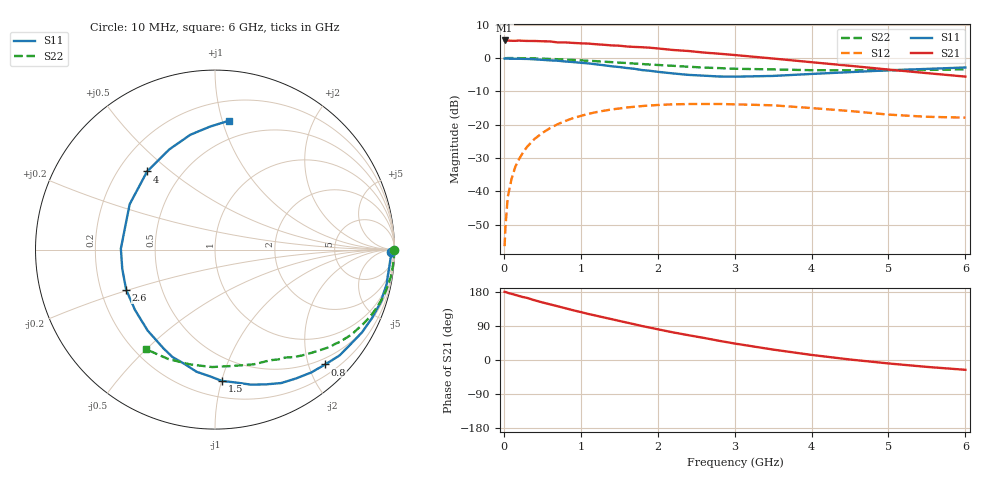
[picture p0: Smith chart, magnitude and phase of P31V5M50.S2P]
! SIEMENS Small Signal Semiconductors
! BFP181
! Si NPN RF Bipolar Junction Transistor in SOT143
! VCE = 1.5 V  IC = 0.5 mA
! Common Emitter S-Parameters:  March  1996
# GHz  S  MA  R  50
!  f  S11  S21  S12  S22
! GHz  MAG  ANG  MAG  ANG  MAG  ANG  MAG  ANG
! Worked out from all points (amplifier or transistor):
!   36 points, 10 MHz to 6 GHz, reference 50 ohm
!   highest |S21| = 5.3 dB at 10 MHz (marker M1)
!   |S21| within 3 dB of that: start of sweep to 2.291 GHz
!   unconditionally stable (mu >= 1): 3.69 GHz to end of sweep
!   at 250 MHz: K = 0.08, MSG = 16.8 dB, |S12| = -28.3 dB
!   at 1.4 GHz: K = 0.44, MSG = 9.6 dB, |S12| = -15.4 dB
!   at 6 GHz: K = 1.50, MAG = 2.0 dB, |S12| = -17.9 dB
!   S11 on the Smith chart (normalised r, x): 10 MHz: 75, -48; 800 MHz: 0.38, -2.29; 1.5 GHz: 0.32, -1.00; 2.6 GHz: 0.31, -0.20; 4 GHz: 0.32, +0.42; 6 GHz: 0.35, +1.05
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0.01  0.9812 -0.7  1.834 179.8  0.0015 89.0  0.9995 -0.2
0.02  0.9871 -1.4  1.833 179.6  0.0028 93.1  0.9925 -0.6
0.05  0.9793 -2.8  1.826 177.3  0.0081 89.5  0.998 -1.5
0.1  0.9757 -5.8  1.814 174.6  0.0153 85.8  0.9978 -2.8
0.15  0.9738 -8.7  1.811 171.8  0.0235 83.8  0.996 -4.2
0.25  0.9703 -14.5  1.813 166.0  0.0383 80.1  0.9928 -7.2
0.3  0.9694 -17.4  1.804 164.0  0.0462 77.7  0.992 -8.5
0.4  0.9546 -23.4  1.801 157.6  0.061 73.6  0.9854 -11.3
0.6  0.9214 -34.9  1.773 146.9  0.0886 65.2  0.9688 -16.9
0.8  0.8868 -46.2  1.712 136.6  0.1135 57.5  0.9475 -22.0
1.1  0.83 -63.6  1.646 121.4  0.1451 46.4  0.9081 -29.3
1.5  0.7326 -87.0  1.53 103.2  0.1747 33.0  0.8511 -38.1
1.9  0.6434 -111.7  1.427 85.4  0.1936 21.6  0.797 -45.5
2.2  0.5867 -129.8  1.319 72.9  0.2018 14.2  0.7635 -50.6
2.6  0.5431 -155.7  1.207 58.3  0.2041 5.3  0.7179 -56.9
3  0.5245 179.4  1.109 43.5  0.2017 -3.3  0.6896 -63.3
3.5  0.5384 152.0  0.982 27.5  0.1951 -11.4  0.6748 -71.3
4  0.5767 131.0  0.865 13.4  0.1773 -17.6  0.6562 -80.9
4.5  0.6136 114.5  0.764 1.3  0.1601 -22.3  0.6546 -91.4
5  0.6545 102.1  0.671 -9.1  0.1414 -23.2  0.6545 -102.2
5.5  0.686 92.3  0.593 -18.2  0.1312 -19.5  0.663 -113.3
6  0.7212 84.0  0.526 -25.9  0.1273 -15.2  0.6751 -124.6
